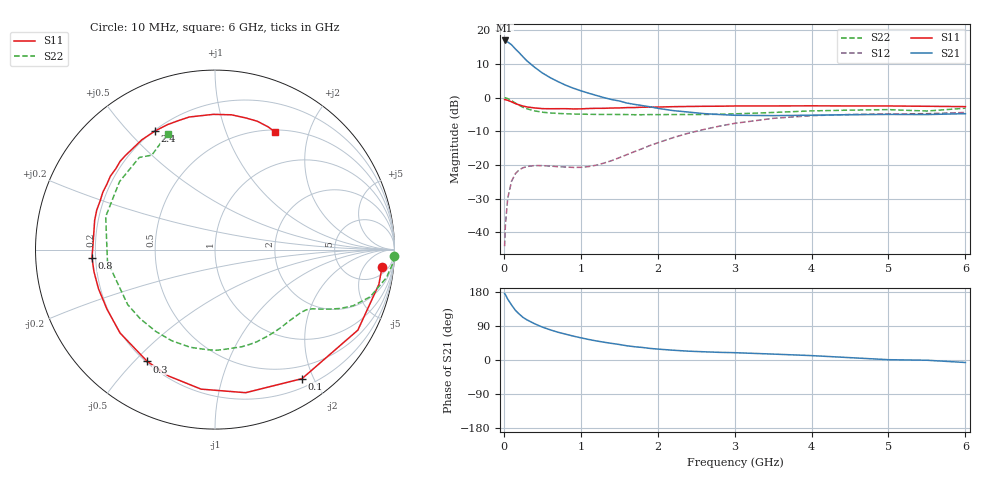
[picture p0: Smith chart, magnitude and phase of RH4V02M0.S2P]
! SIEMENS Small Signal Semiconductors
! BFR106
! Si NPN RF Bipolar Junction Transistor in SOT23
! VCE = 4 V  IC = 2 mA
! Common Emitter S-Parameters:  August  1996
# GHz  S  MA  R  50
!  f  S11  S21  S12  S22
! GHz  MAG  ANG  MAG  ANG  MAG  ANG  MAG  ANG
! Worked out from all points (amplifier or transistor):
!   36 points, 10 MHz to 6 GHz, reference 50 ohm
!   highest |S21| = 17.0 dB at 10 MHz (marker M1)
!   |S21| within 3 dB of that: start of sweep to 170.9 MHz
!   unconditionally stable (mu >= 1): 791 MHz to 1.873 GHz; 3.822 GHz to end of sweep
!   at 250 MHz: K = 0.32, MSG = 16.5 dB, |S12| = -20.8 dB
!   at 1.4 GHz: K = 1.27, MAG = 6.0 dB, |S12| = -18.7 dB
!   at 6 GHz: K = 1.02, MAG = -1.1 dB, |S12| = -4.4 dB
!   S11 on the Smith chart (normalised r, x): 10 MHz: 9, -14; 100 MHz: 0.32, -1.84; 300 MHz: 0.21, -0.55; 800 MHz: 0.19, -0.03; 2.4 GHz: 0.20, +0.60; 6 GHz: 0.52, +1.50
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0.01  0.9359 -5.9  7.093 175.5  0.0062 89.6  0.9997 -2.1
0.02  0.9334 -12.0  7.024 172.5  0.0126 82.6  0.9964 -4.0
0.05  0.9137 -29.4  6.732 160.8  0.0317 74.3  0.9677 -9.3
0.1  0.8672 -56.0  6.123 145.3  0.0571 61.1  0.9041 -16.9
0.15  0.8153 -77.9  5.301 131.2  0.0742 49.6  0.831 -22.1
0.2  0.7813 -95.7  4.657 121.2  0.0848 42.3  0.7704 -25.2
0.25  0.7504 -110.1  4.043 112.3  0.0907 36.5  0.7179 -27.5
0.3  0.7284 -121.2  3.533 106.0  0.0948 32.8  0.6838 -29.0
0.4  0.7042 -138.7  2.833 95.6  0.0979 27.8  0.6366 -31.2
0.5  0.6873 -151.2  2.334 86.9  0.0977 25.8  0.6084 -33.5
0.6  0.6848 -161.4  1.993 79.8  0.0963 25.7  0.593 -36.3
0.8  0.687 -176.2  1.54 68.3  0.0932 29.8  0.5762 -42.5
1.1  0.6901 166.3  1.168 54.3  0.0945 44.5  0.566 -53.5
1.6  0.7122 144.9  0.832 37.5  0.1423 66.5  0.5616 -74.7
2.2  0.7352 123.7  0.643 25.8  0.2545 67.4  0.5615 -104.1
2.4  0.7403 116.9  0.611 23.3  0.2967 64.3  0.5621 -115.4
3  0.7526 101.0  0.548 19.3  0.4152 51.2  0.575 -147.8
3.5  0.7536 90.7  0.541 15.6  0.4927 39.1  0.6029 -173.7
4.5  0.7533 76.6  0.558 6.2  0.5627 17.1  0.653 144.5
5  0.7531 71.8  0.564 0.8  0.5742 8.8  0.6645 129.4
5.5  0.745 66.5  0.561 -0.6  0.5784 4.8  0.6332 123.8
6  0.7362 63.1  0.579 -6.6  0.6031 -3.1  0.6979 112.2
